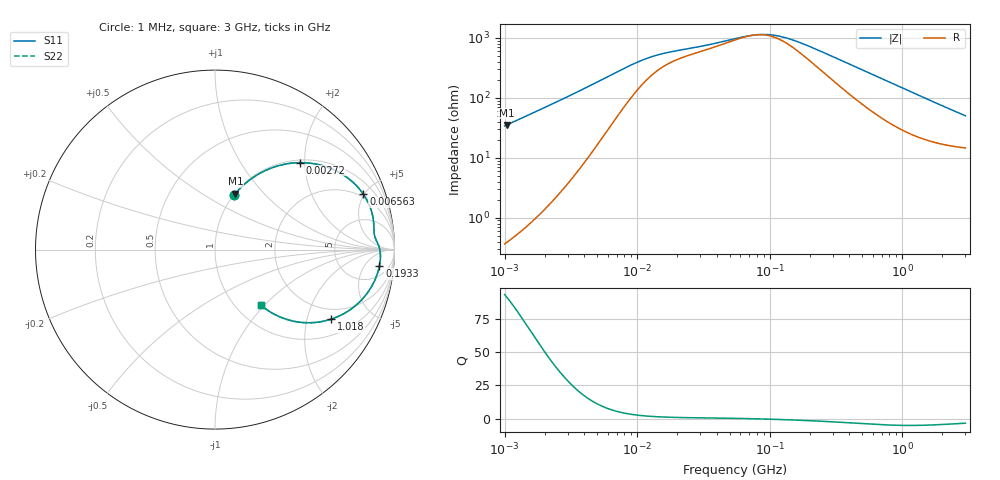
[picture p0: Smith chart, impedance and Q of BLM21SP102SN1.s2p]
! BLM21SP102SN1
# Hz S RI R 50
!Freq.(Hz) S11(Real) S11(Imag) S21(Real) S21(Imag) S12(Real) S12(Imag) S22(Real) S22(Imag)
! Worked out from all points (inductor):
!   401 points, 1 MHz to 3 GHz, reference 50 ohm
!   read as one part in series: L = 5.42 uH near 1.041 MHz
!   highest Q = 90.9 at 1.041 MHz (marker M1), where L = 5.41 uH
!   self-resonance near 78.3 MHz
!   S11 on the Smith chart (normalised r, x): 1 MHz: 1.01, +0.68; 2.72 MHz: 1.06, +1.89; 6.563 MHz: 1.77, +4.94; 193.3 MHz: 10, -12; 1.018 GHz: 1.57, -2.82; 3 GHz: 1.29, -0.96
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1000000  0.1061 0.3026  0.8939 -0.3026  0.8939 -0.3026  0.1061 0.3026
1040844  0.1139 0.3122  0.8861 -0.3122  0.8861 -0.3122  0.1139 0.3122
1649378  0.245 0.4222  0.755 -0.4222  0.755 -0.4222  0.245 0.4222
2139570  0.3551 0.4679  0.6449 -0.4679  0.6449 -0.4679  0.3551 0.4679
2720446  0.4738 0.4844  0.5262 -0.4844  0.5262 -0.4844  0.4738 0.4844
3823119  0.6431 0.453  0.3569 -0.453  0.3569 -0.453  0.6431 0.453
5059610  0.7564 0.3858  0.2436 -0.3858  0.2436 -0.3858  0.7564 0.3858
6563319  0.827 0.308  0.173 -0.308  0.173 -0.308  0.827 0.308
1.061086e7  0.8798 0.1804  0.1202 -0.1804  0.1202 -0.1804  0.8798 0.1804
1.461624e7  0.8855 0.1253  0.1145 -0.1253  0.1145 -0.1253  0.8855 0.1253
5.477226e7  0.9102 0.0267  0.0898 -0.0267  0.0898 -0.0267  0.9102 0.0267
7.697298e7  0.9179 0.00138  0.0821 -0.00138  0.0821 -0.00138  0.9179 0.00138
1.018679e8  0.9213 -0.0225  0.0787 0.0225  0.0787 0.0225  0.9213 -0.0225
1.348146e8  0.9215 -0.0498  0.0785 0.0498  0.0785 0.0498  0.9215 -0.0498
1.93289e8  0.9162 -0.0913  0.0838 0.0913  0.0838 0.0913  0.9162 -0.0913
2.094008e8  0.9139 -0.1018  0.0861 0.1018  0.0861 0.1018  0.9139 -0.1018
4.480278e8  0.8563 -0.2311  0.1437 0.2311  0.1437 0.2311  0.8563 -0.2311
8.005644e8  0.7289 -0.3505  0.2711 0.3505  0.2711 0.3505  0.7289 -0.3505
1.017911e9  0.6467 -0.3877  0.3533 0.3877  0.3533 0.3877  0.6467 -0.3877
1.645649e9  0.4541 -0.402  0.5459 0.402  0.5459 0.402  0.4541 -0.402
2.312676e9  0.3303 -0.3602  0.6697 0.3602  0.6697 0.3602  0.3303 -0.3602
3e9  0.2578 -0.3112  0.7422 0.3112  0.7422 0.3112  0.2578 -0.3112
